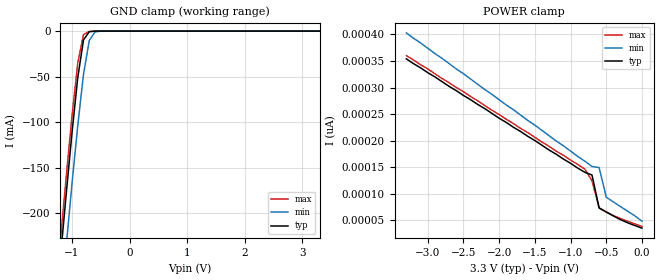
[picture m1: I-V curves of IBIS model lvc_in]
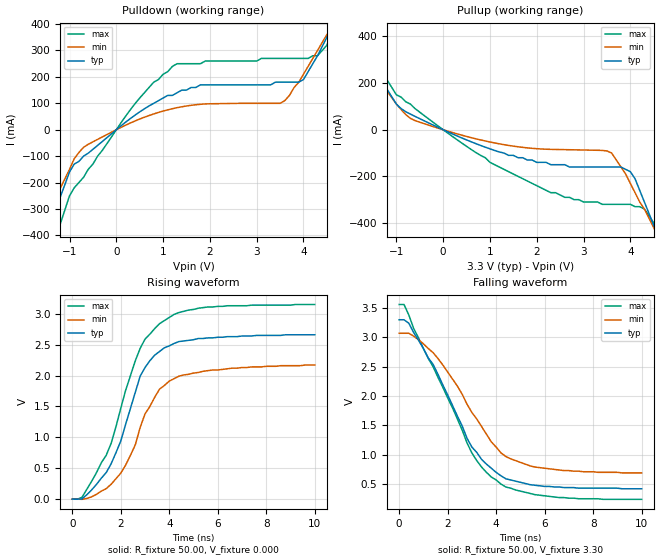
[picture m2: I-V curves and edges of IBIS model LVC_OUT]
| IBIS file THS5661.ibs created Dave Fletcher of Texas Instruments
[IBIS ver]   2.1
[File name]   ths5661.ibs
[File Rev]   1.0
[Date]   01/25/2001
[Source]   Texas Instruments - BWA
[Notes]
[Disclaimer]
[Copyright]
|   Component THS5661
[Component]   THS5661
[Manufacturer]   Texas Instruments
[Package]
|PHP
| variable   typ   min   max
R_pkg   6.50m   NA   NA
L_pkg   3.20nH   NA   NA
C_pkg   4.00pF   NA   NA
[Pin]  signal_name   model_name   R_pin   L_pin   C_pin
1   D11   lvc_in
2   D10   lvc_in
3   D9   lvc_in
4   D8   lvc_in
5   D7   lvc_in
6   D6   lvc_in
7   D5   lvc_in
8   D4   lvc_in
9   D3   lvc_in
10   D2   lvc_in
11   D1   lvc_in
12   D0   lvc_in
13   NC   NC
14   NC   NC
15   SLEEP   NC
16   EXTLO   NC
17   EXTIO   NC
18   BIASJ   NC
19   COMP1   NC
20   AGND   GND
21   IOUT2   LVC_OUT
22   IOUT1   LVC_OUT
23   COMP2   NC
24   AVDD   POWER
25   MODE   NC
26   DGND   GND
27   DVDD   POWER
28   CLK   lvc_in
| Models and submodels in the file (2): lvc_in (Input), LVC_OUT (Output)
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|   Model lvc_in
[Model]   lvc_in
Model_type   Input
Vinl =  0.800V
Vinh =  2.000V
|   typ   min   max
C_comp   3.00pF   NA   NA
|   typ   max   min
[Temperature Range]   25.00   100.00   0.000
[Voltage Range]   3.30V   3.00V   3.60V
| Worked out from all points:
|   GND clamp passes 1 mA (typ) near -0.70 V on its own axis
[GND_clamp]
| voltage   I(typ)   I(min)   I(max)
-3.3V     -1.806A    -1.858A    -1.789A
-1.2V     -248mA     -306mA     -229mA
-1.1V     -179mA     -236mA     -160mA
-1V       -112mA     -168mA     -93.56mA
-900mV    -51.39mA   -104mA     -35.36mA
-800mV    -9.697mA   -47.7mA    -3.786mA
-700mV    -714uA     -10.4mA    -348uA
-600mV    -52.42uA   -951uA     -8.225uA
-500mV    -126nA     -30.48uA   -10.89nA
3.3V      34.69pA    75.27pA    23pA
[POWER_clamp]
| voltage   I(typ)   I(min)   I(max)
-3.3V     354pA      403pA      360pA
-800mV    140pA      161pA      146pA
-700mV    135pA      151pA      124pA
-600mV    72.75pA    149pA      72.79pA
-500mV    65.09pA    93.05pA    65.39pA
-300mV    50.77pA    75.27pA    52.78pA
0V        34.68pA    47.91pA    37.83pA
|   Model LVC_OUT
[Model]   LVC_OUT
Model_type   Output
Polarity   Inverting
Vmeas =   1.50V
Cref =  50.00pF
Rref =   0.50k
C_comp   5.00pF   5.00pF   5.00pF
[Temperature Range]   25.00   85.00   -40.00
[Voltage Range]   3.30V   3.00V   3.60V
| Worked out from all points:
|   slope of the pulldown table from 0 to 0.495 V, typ, clamps not added: 7.4 ohm
|   slope of the pullup table from 0 to 0.495 V, typ, clamps not added: 11.4 ohm
|   rising waveform, R_fixture 50.00, V_fixture 0.000: 20-80 % time 1.45ns typ, 1.51ns min, 1.64ns max; typ from 0 V to 2.66 V
|   falling waveform, R_fixture 50.00, V_fixture 3.30: 20-80 % time 2.17ns typ, 2.24ns min, 2.29ns max; typ from 3.3 V to 0.42 V
[Pulldown]
| voltage   I(typ)   I(min)   I(max)
-3.3V     -1.33A     -1.04A     -1.93A
-1.7V     -500mA     -410mA     -670mA
-1.5V     -400mA     -330mA     -520mA
-900mV    -130mA     -110mA     -220mA
-600mV    -88.67mA   -55.17mA   -150mA
500mV     67.5mA     40.46mA    120mA
1.3V      140mA      83.53mA    250mA
3.5V      180mA      100mA      270mA
4V        190mA      210mA      270mA
4.3V      280mA      300mA      280mA
4.7V      420mA      410mA      410mA
6.6V      1.12A      980mA      1.32A
[Pullup]
| voltage   I(typ)   I(min)   I(max)
-3.3V     910mA      770mA      1.14A
-2.3V     560mA      480mA      680mA
-1.9V     410mA      360mA      490mA
-1V       110mA      110mA      150mA
-800mV    77.22mA    64.82mA    120mA
1V        -81.97mA   -52.55mA   -140mA
2.3V      -150mA     -84.19mA   -270mA
3.6V      -160mA     -100mA     -320mA
4V        -180mA     -230mA     -320mA
4.5V      -410mA     -420mA     -400mA
4.7V      -510mA     -500mA     -540mA
6.6V      -1.51A     -1.25A     -2.04A
[Ramp]
| variable   typ   min   max
dV/dt_r   1.94/1.12n   1.74/0.95n   2.13/1.45n
dV/dt_f   1.95/1.77n   1.76/1.59n   2.14/2.05n
R_load = 0.50k
[Rising Waveform]
R_fixture = 50.00
V_fixture = 0.000
| time   V(typ)   V(min)   V(max)
0s        0V         0V         0V
400ps     3.71mV     -3.16mV    28.86mV
1.4ns     430mV      170mV      710mV
2ns       940mV      420mV      1.47V
2.6ns     1.73V      880mV      2.24V
2.8ns     1.99V      1.16V      2.44V
3.6ns     2.39V      1.78V      2.84V
4.4ns     2.55V      1.99V      3.02V
5.4ns     2.6V       2.07V      3.1V
10ns      2.66V      2.17V      3.15V
[Falling Waveform]
R_fixture = 50.00
V_fixture = 3.30
| time   V(typ)   V(min)   V(max)
0s        3.3V       3.07V      3.56V
200ps     3.3V       3.07V      3.56V
400ps     3.24V      3.07V      3.38V
1.4ns     2.54V      2.74V      2.5V
2.4ns     1.66V      2.17V      1.61V
3ns       1.13V      1.72V      1.03V
3.8ns     770mV      1.22V      620mV
4.4ns     590mV      970mV      450mV
5.6ns     480mV      790mV      320mV
10ns      420mV      690mV      240mV
